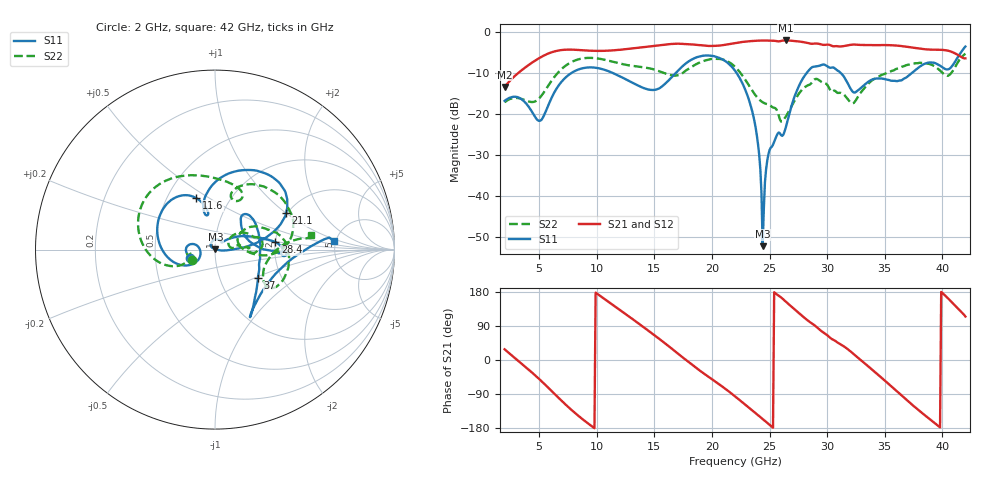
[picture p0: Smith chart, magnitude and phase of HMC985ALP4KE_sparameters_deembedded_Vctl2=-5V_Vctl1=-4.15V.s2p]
!s2p File: Measurements: S11, S21, S12, S22
# GHz S dB R 50.0
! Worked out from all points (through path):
!   401 points, 2 GHz to 42 GHz, reference 50 ohm
!   highest |S21| = -2.07 dB at 26.4 GHz (marker M1); lowest = -13.4 dB at 2 GHz (marker M2)
!   lowest |S11| = -52.3 dB at 24.4 GHz (marker M3), VSWR 1.00, Z = 50.2 + j0.115 ohm
!   |S11| at or under -10 dB: start of sweep to 7.808 GHz; 22.13 GHz to 28.23 GHz (6.092 GHz wide, 24.2 % of centre); 31.18 GHz to 37.36 GHz (6.185 GHz wide, 18 % of centre)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
!   |S22| runs from -21.9 to -5.3 dB; largest |S21 - S12| = 0.00074
!   S11 on the Smith chart (normalised r, x): 2 GHz: 0.76, -0.07; 11.6 GHz: 0.69, +0.44; 21.1 GHz: 1.97, +1.01; 28.4 GHz: 2.00, +0.19; 37 GHz: 1.52, -0.53; 42 GHz: 4.82, +0.80
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2  -16.83 -161.9  -13.45 28.2  -13.45 28.2  -17.16 -155.9
5  -21.71 -173.1  -6.39 -50.1  -6.39 -50.1  -16.21 -160.0
6.3  -14.84 -150.7  -4.77 -88.3  -4.77 -88.4  -11.06 -161.6
8.7  -8.90 150.2  -4.45 -154.6  -4.45 -154.6  -6.49 151.3
11.6  -10.28 110.2  -4.45 140.9  -4.45 140.9  -7.42 103.5
13.6  -13.11 101.0  -3.85 97.1  -3.86 97.1  -8.46 75.9
15.4  -13.80 105.6  -3.25 56.3  -3.25 56.3  -9.55 62.6
17.9  -7.32 79.9  -2.95 -3.7  -2.95 -3.7  -9.12 72.2
21.1  -7.01 27.2  -3.14 -74.6  -3.14 -74.6  -6.88 16.0
22  -9.44 16.7  -2.71 -95.8  -2.71 -95.8  -8.50 0.6
23.6  -20.62 -0.2  -2.18 -135.6  -2.18 -135.6  -14.76 -3.7
24  -27.44 -7.0  -2.12 -145.6  -2.12 -145.6  -16.22 2.0
24.4  -52.30 28.0  -2.09 -155.8  -2.09 -155.7  -17.16 7.7
25  -28.82 133.0  -2.12 -171.0  -2.12 -171.0  -17.84 11.1
26.4  -23.39 43.4  -2.07 154.3  -2.07 154.3  -20.70 33.0
28.4  -9.40 7.1  -2.75 102.3  -2.75 102.3  -12.95 18.3
28.7  -8.59 2.0  -2.88 96.1  -2.89 96.2  -12.22 16.5
32.5  -14.64 33.9  -3.09 10.3  -3.09 10.3  -16.63 29.2
35.4  -11.76 18.7  -3.22 -65.1  -3.21 -65.1  -9.78 19.4
37  -10.82 -33.7  -3.64 -108.2  -3.64 -108.1  -8.02 4.9
39.8  -8.22 -56.6  -4.34 -177.7  -4.34 -177.7  -9.41 -34.7
42  -3.55 4.0  -6.43 114.8  -6.43 114.8  -5.29 8.7
